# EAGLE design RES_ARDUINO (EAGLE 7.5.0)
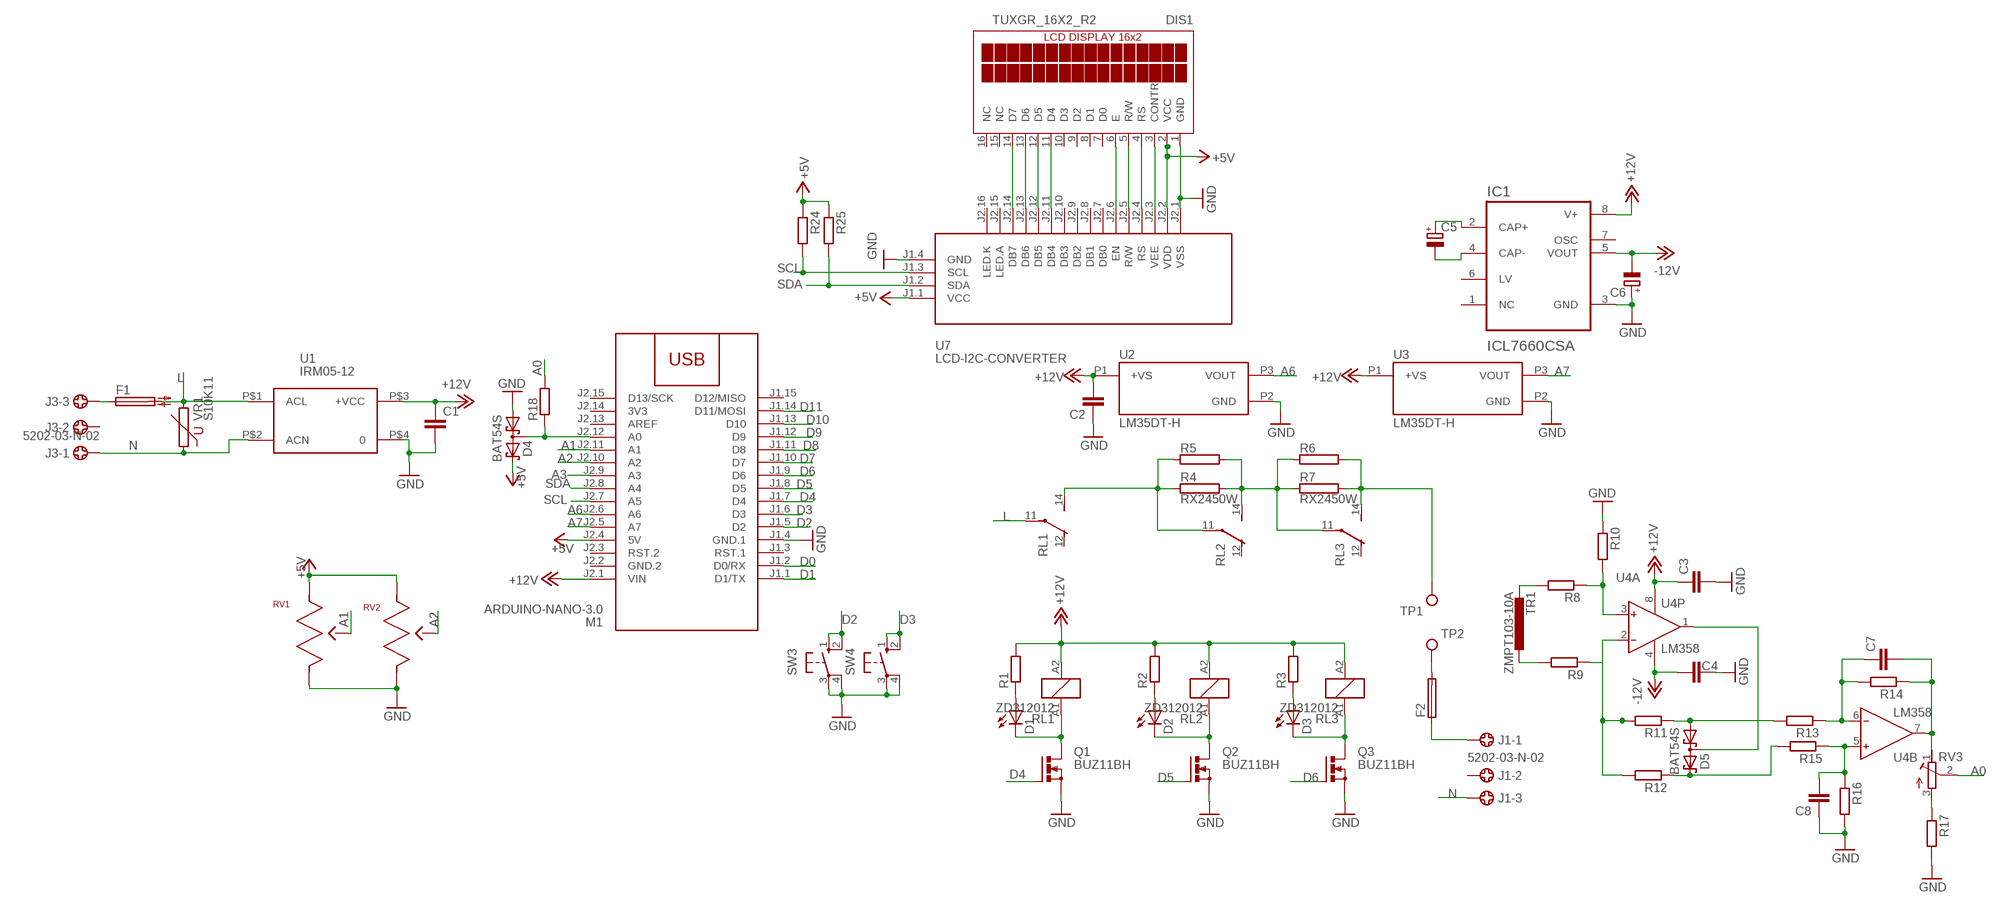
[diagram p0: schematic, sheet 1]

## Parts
C1  C-EUC1206  [C1206]
C2  C-EUC1206  [C1206]
C3  C-EUC1206  [C1206]
C4  C-EUC1206  [C1206]
C5  CPOL-EUSMCB  [SMC_B]
C6  CPOL-EUSMCB  [SMC_B]
C7  C-EUC1206  [C1206]
C8  C-EUC1206  [C1206]
D1  LED5MM  [LED5MM]
D2  LED5MM  [LED5MM]
D3  LED5MM  [LED5MM]
D4  BAT54S  [SOT23]
D5  BAT54S  [SOT23]
DIS1  TUXGR_16X2_R2  [TUXGR_16X2_R2]
F1  SH22,5A  [SH22,5A]
F2  SH22,5A  [SH22,5A]
IC1  ICL7660CSA  [SOIC127P600X175-8N]
J1  5202-03-N-02  [5202-03-N-02]
J3  5202-03-N-02  [5202-03-N-02]
M1  ARDUINO-NANO-3.0  [ARDUINO-NANO-3.0]
Q1  BUZ11BH  [TO220BH]
Q2  BUZ11BH  [TO220BH]
Q3  BUZ11BH  [TO220BH]
R1  R-EU_R1206  [R1206]
R2  R-EU_R1206  [R1206]
R3  R-EU_R1206  [R1206]
R4  RX2450W  [RX2450W]
R5  RX2450W  [RX2450W]
R6  RX2450W  [RX2450W]
R7  RX2450W  [RX2450W]
R8  R-EU_R1206  [R1206]
R9  R-EU_R1206  [R1206]
R10  R-EU_R1206  [R1206]
R11  R-EU_R1206  [R1206]
R12  R-EU_R1206  [R1206]
R13  R-EU_R1206  [R1206]
R14  R-EU_R1206  [R1206]
R15  R-EU_R1206  [R1206]
R16  R-EU_R1206  [R1206]
R17  R-EU_R1206  [R1206]
R18  R-EU_R1206  [R1206]
R24  R-EU_R1206  [R1206]
R25  R-EU_R1206  [R1206]
RL1  ZD312012  [ZD1]
RL2  ZD312012  [ZD1]
RL3  ZD312012  [ZD1]
RV1  PTV09A-4025F-A103  [PTV09]
RV2  PTV09A-4025F-A103  [PTV09]
RV3  R-TRIMM-3386-F  [R-TRIMM-3386F]
SW3  10-XX  [B3F-10XX]
SW4  10-XX  [B3F-10XX]
TP1  TPPAD1-20Y  [P1-20Y]
TP2  TPPAD1-20Y  [P1-20Y]
TR1  ZMPT103-10A  [ZMPT103-10A]
U1  IRM05-12  [IRM05-12]
U2  LM35DT-H  [LM35DT-H]
U3  LM35DT-H  [LM35DT-H]
U4  LM358  AD8042N  [DIL08]
U7  LCD-I2C-CONVERTER  [LCD-I2C-CONVERTER]
VR1  S10K11  [S10K11]

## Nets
+5V: D4.2(C2) DIS1.2(VCC) M1.J2.4(5V) R24.1 R25.1 RV1.1 RV2.1 U7.J1.1(VCC) U7.J2.2(VDD)
+12V: C1.1 C2.2 C3.1 IC1.8(V+) M1.J2.1(VIN) R1.2 R2.2 R3.2 RL1.A2 RL2.A2 RL3.A2 U1.P$3(+VCC) U2.P1(+VS) U3.P1(+VS) U4.8(P:V+)
-12V: C4.1 C6.- IC1.5(VOUT) U4.4(P:V-)
A0: R18.2 RV3.2(S)
A1: M1.J2.11(A1) RV1.2
A2: M1.J2.10(A2) RV2.2
A3: M1.J2.9(A3)
A6: M1.J2.6(A6) U2.P3(VOUT)
A7: M1.J2.5(A7) U3.P3(VOUT)
D0: M1.J1.2(D0/RX)
D1: M1.J1.1(D1/TX)
D2: M1.J1.5(D2) SW3.1(S) SW3.2(S1)
D3: M1.J1.6(D3) SW4.1(S) SW4.2(S1)
D4: M1.J1.7(D4) Q1.G
D5: M1.J1.8(D5) Q2.G
D6: M1.J1.9(D6) Q3.G
D7: M1.J1.10(D7)
D8: M1.J1.11(D8)
D9: M1.J1.12(D9)
D10: M1.J1.13(D10)
D11: M1.J1.14(D11/MOSI)
GND: C1.2 C2.1 C3.2 C4.2 C6.+ C8.1 D4.1(A1) DIS1.1(GND) IC1.3(GND) M1.J1.4(GND.1) Q1.S Q2.S Q3.S R10.1 R16.2 R17.2 RV1.3 RV2.3 SW3.3(P) SW3.4(P1) SW4.3(P) SW4.4(P1) U1.P$4 U2.P2(GND) U3.P2(GND) U7.J1.4(GND) U7.J2.1(VSS)
L: F1.2 RL1.11(2:P) U1.P$1(ACL) VR1.2
N: J1.3 J3.1 U1.P$2(ACN) VR1.1
N$1: DIS1.14(D7) U7.J2.14(DB7)
N$2: DIS1.13(D6) U7.J2.13(DB6)
N$3: DIS1.12(D5) U7.J2.12(DB5)
N$4: DIS1.11(D4) U7.J2.11(DB4)
N$5: DIS1.6(E) U7.J2.6(EN)
N$6: DIS1.5(R/W) U7.J2.5(R/W)
N$7: DIS1.4(RS) U7.J2.4(RS)
N$8: F1.1 J3.3
N$9: D2.A R2.1
N$10: DIS1.3(CONTR) U7.J2.3(VEE)
N$12: D1.K(C) Q1.D RL1.A1
N$13: D2.K(C) Q2.D RL2.A1
N$14: D3.K(C) Q3.D RL3.A1
N$15: R4.P$1 R5.P$1 RL1.14(2:S) RL2.11(2:P)
N$16: R4.P$2 R5.P$2 R6.P$1 R7.P$1 RL2.14(2:S) RL3.11(2:P)
N$17: D1.A R1.1
N$18: D3.A R3.1
N$19: F2.2 TP2.TP
N$20: R6.P$2 R7.P$2 RL3.14(2:S) TP1.TP
N$21: F2.1 J1.1
N$22: R8.2 TR1.P$1
N$23: R9.2 TR1.P$2
N$24: R8.1 R10.2 U4.3(A:IN+)
N$25: C5.+ IC1.2(CAP+)
N$26: C5.- IC1.4(CAP-)
N$27: R9.1 R11.2 R12.2 U4.2(A:IN-)
N$28: D5.1(A1) R11.1 R13.2
N$29: D5.2(C2) R12.1 R15.2
N$30: D5.3(C1A2) U4.1(A:OUT)
N$31: C7.1 R13.1 R14.2 U4.6(B:IN-)
N$32: R17.1 RV3.3(E)
N$33: C8.2 R15.1 R16.1 U4.5(B:IN+)
N$34: D4.3(C1A2) M1.J2.12(A0) R18.1
N$35: C7.2 R14.1 RV3.1(A) U4.7(B:OUT)
SCL: M1.J2.7(A5) R24.2 U7.J1.3(SCL)
SDA: M1.J2.8(A4) R25.2 U7.J1.2(SDA)
Unconnected: DIS1.7(D0) DIS1.8(D1) DIS1.9(D2) DIS1.10(D3) DIS1.15(NC) DIS1.16(NC) IC1.1(NC) IC1.6(LV) IC1.7(OSC) J1.2 J3.2 M1.J1.3(RST.1) M1.J1.15(D12/MISO) M1.J2.3(RST.2) M1.J2.13(AREF) M1.J2.15(D13/SCK) RL1.12(2:O) RL2.12(2:O) RL3.12(2:O) U7.J2.7(DB0) U7.J2.8(DB1) U7.J2.9(DB2) U7.J2.10(DB3) U7.J2.15(LED.A) U7.J2.16(LED.K)

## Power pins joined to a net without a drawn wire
3V3: M1.J2.14(3V3)
GND.2: M1.J2.2(GND.2)

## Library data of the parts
C1-C4 C7 C8 = rcl:C-EU: CAPACITOR, European symbol
C5 C6 = rcl:CPOL-EU: POLARIZED CAPACITOR, European symbol
D1-D3 = led:LED: LED
D4 D5 = diode:BAT54S: Schottky Diodes Pin connection corrected 2011-05-04 Source: Fairchild .. BAT54.pdf
DIS1 = display-lcd:TUXGR_16X2_R2: Tuxgraphics LCD display 16x2 characters reflective, without background light Source: tuxgr_12x2_r2.pdf; OC_FARNELL: unknown; OC_NEWARK: unknown
F1 F2 = fuse:SH22,5A: FUSE HOLDER; MPN: 0031.7701.11; OC_FARNELL: unknown; OC_NEWARK: 04F1224
IC1 = ICL7660CSA:ICL7660CSA: Check availability; AVAILABILITY: In Stock; CHECK_PRICES: https://www.snapeda.com/parts/ICL7660CSA/Analog+Devices/view-part/?ref=eda; DESCRIPTION: Charge Pump Switching Regulator IC Positive or Negative Fixed -Vin, nVin, Vin/2 1 Output 20mA 8-SOIC (0.154, 3.90mm Width); MF: Analog Devices; MP: ICL7660CSA; PACKAGE: SOIC-8 Maxim; PRICE: None; SNAPEDA_LINK: https://www.snapeda.com/parts/ICL7660CSA/Analog+Devices/view-part/?ref=snap
J1 J3 = con-ebyelectro:5202-03-N-02: Barrier Blocks Sreies 5202 Source: http://www.ebyelectro.com/PDF/5202-XX-N-02.pdf; OC_FARNELL: unknown; OC_NEWARK: unknown
M1 = diy-modules:ARDUINO-NANO-3.0: Arduino Nano 3.0 and compatible devices More details available here: https://www.arduino.cc/en/Main/ArduinoBoardNano Click here to find device on ebay.com
Q1-Q3 = transistor-power:BUZ11: N-CHANNEL MOS FET
R1-R3 R8-R18 R24 R25 = rcl:R-EU_: RESISTOR, European symbol
R4-R7 = resistor-power:RX2450W
RL1-RL3 = relay:ZD?1*: Power Relay SCHRACK 1 pole 30 A Source: http://www.schrack.com/.. 5848.pdf; OC_FARNELL: unknown; OC_NEWARK: unknown
RV1 RV2 = PTV09A-4025F-A103:PTV09A-4025F-A103: 10k Ohm 1 Gang Logarithmic Through Hole, Snap In Potentiometer None 1 Turn Carbon 0.05W, 1/20W PC Pins, Board Locks Check availability; AVAILABILITY: In Stock; CHECK_PRICES: https://www.snapeda.com/parts/PTV09A-4025F-A103/Bourns/view-part/?ref=eda; DESCRIPTION: 10k Ohm 1 Gang Logarithmic Through Hole, Snap In Potentiometer None 1.0 Kierros Carbon 0.05W, 1/20W PC Pins, Board Locks; MF: Bourns; MP: PTV09A-4025F-A103; PACKAGE: None; PRICE: None; PURCHASE-URL: https://www.snapeda.com/api/url_track_click_mouser/?unipart_id=1440680&manufacturer=Bourns&part_name=PTV09A-4025F-A103&search_term=ptv09a; SNAPEDA_LINK: https://www.snapeda.com/parts/PTV09A-4025F-A103/Bourns/view-part/?ref=snap
RV3 = rcl:R-TRIMM-3386-F
SW3 SW4 = switch-omron:10-XX: OMRON SWITCH; MPN: B3F-1000; OC_FARNELL: 176432; OC_NEWARK: 36M3542
TP1 TP2 = testpad:TP: Test pad
TR1 = diy-modules:ZMPT103-10A
U1 = acdc:IRM05-12
U2 U3 = LM35DT-H:LM35DT-H
U4 = analog-devices:AD8042: Dual 160 MHz Rail-to-Rail Amplifier Source: http://www.analog.com/static/imported-files/data_sheets/AD8042.pdf; MF: ANALOG DEVICES; MPN: AD8042AN; OC_FARNELL: 1540543; OC_NEWARK: 52F8033
U7 = diy-modules:LCD-I2C-CONVERTER: I2C Bus to 4-Bit Parallel LCD Interface with LED backlight driver
VR1 = varistor:S10K11: VARISTOR

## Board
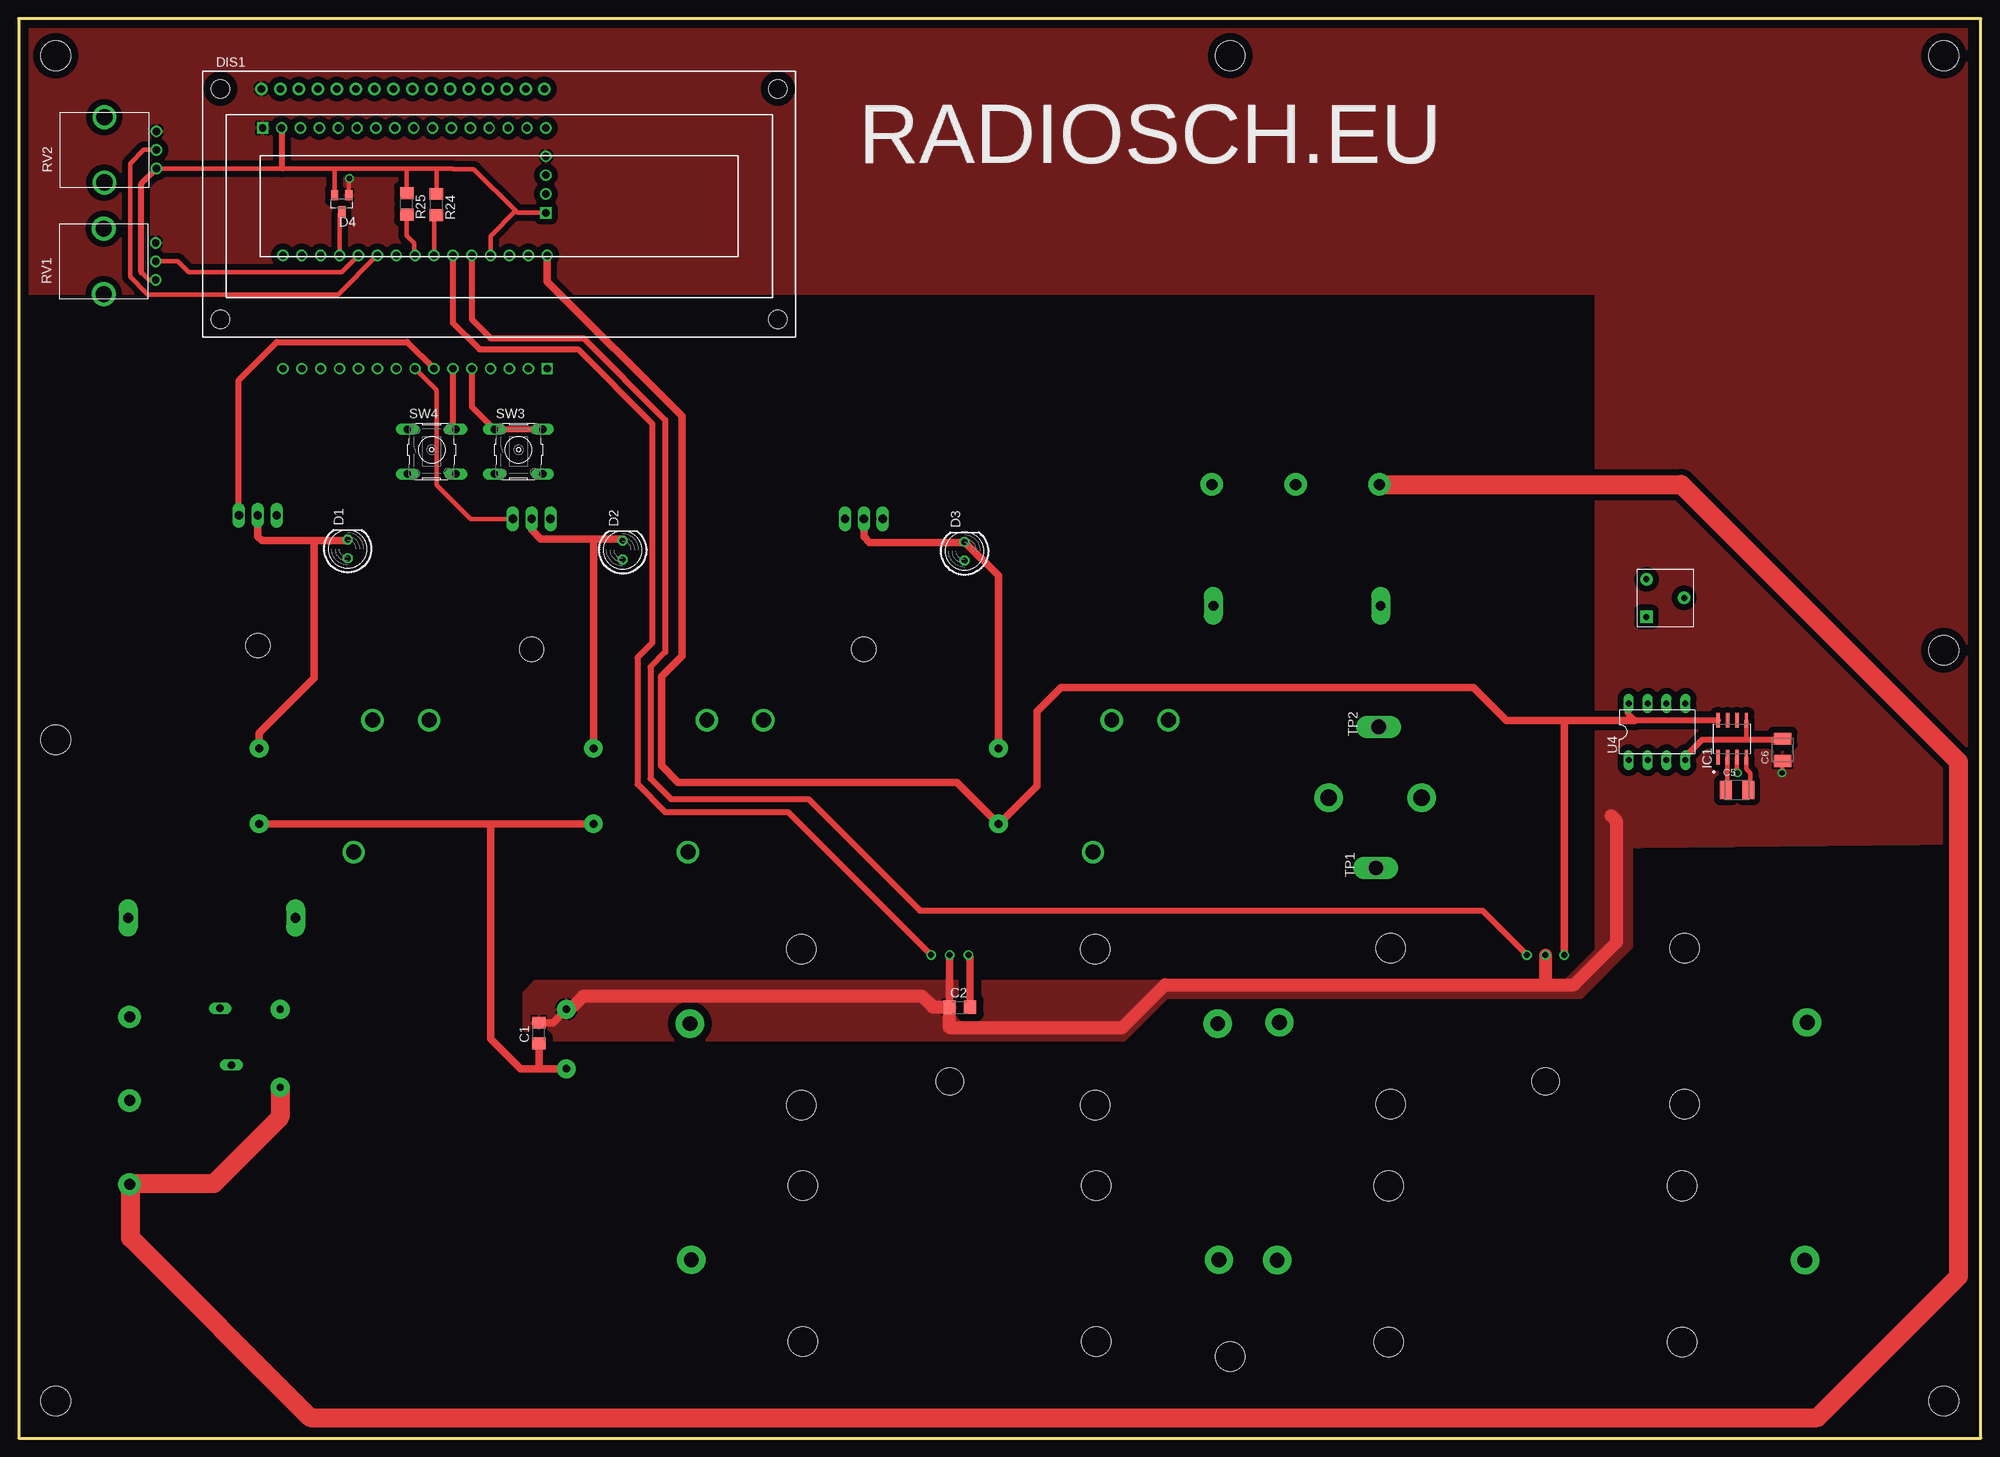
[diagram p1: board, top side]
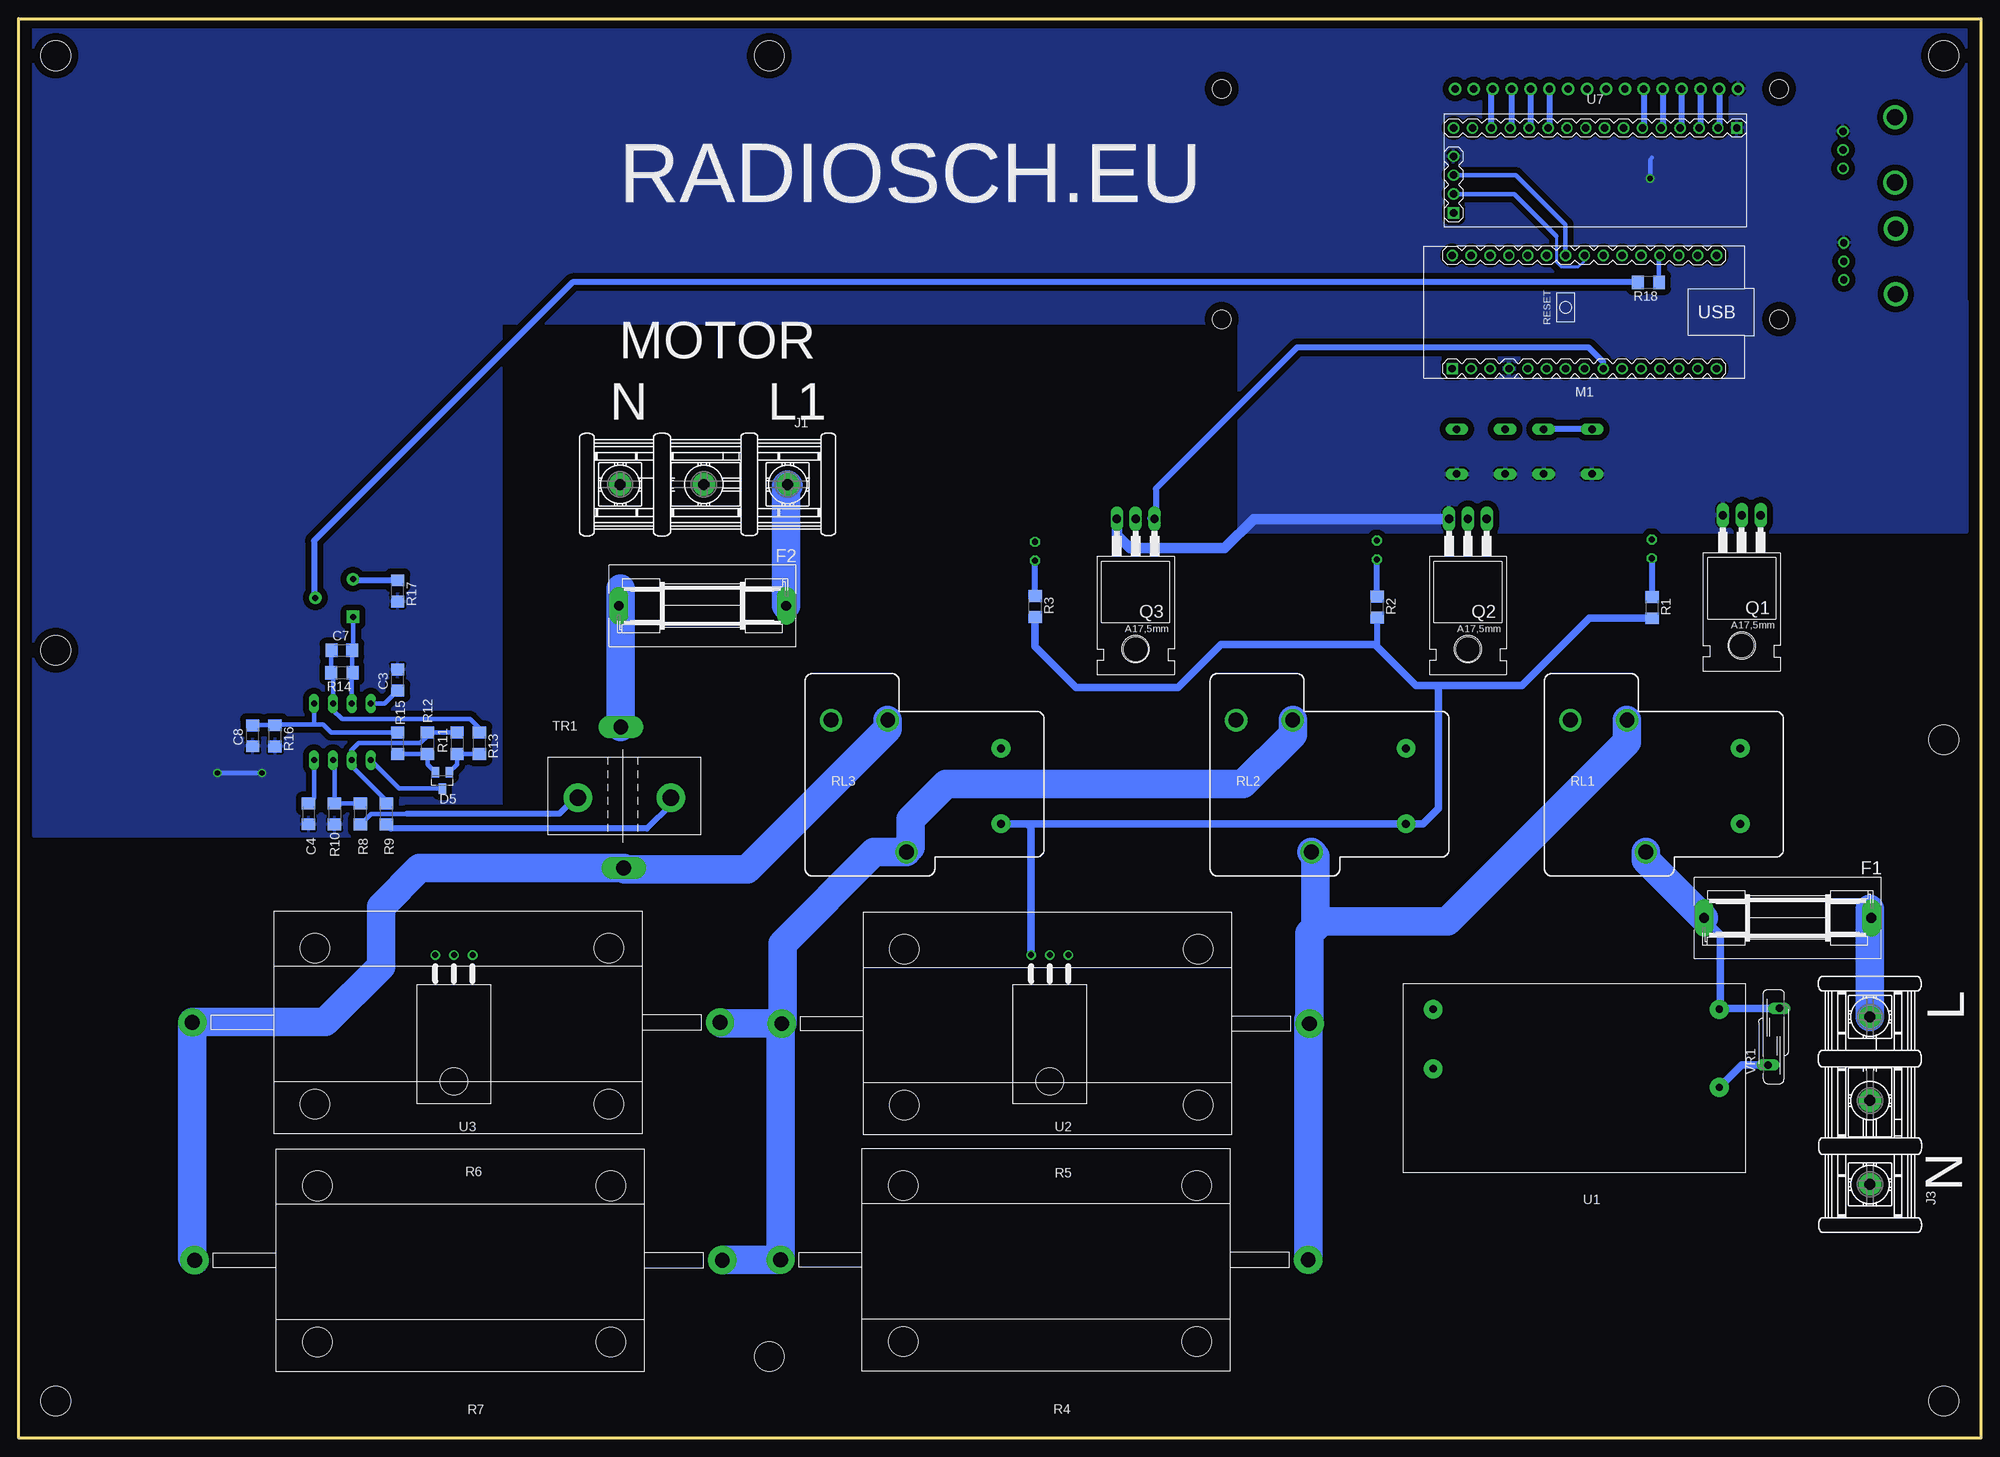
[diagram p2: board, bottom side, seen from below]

Size 264 x 191 mm. Coordinates in mm from the lower left corner, seen from the top.
Outline: 0,0 264,0 264,191 0,191 0,0
Copper layers (1*16): Top 0.035mm / dielectric 1.5mm / Bottom 0.035mm
Design rules "default": minimum track width 10mil, minimum drill 24mil, track to track 8mil, track to pad 8mil, pad to pad 8mil, via to via 8mil, smd to smd 8mil, copper to edge 40mil, drill to drill 8mil, minimum pad ring 10mil, minimum via ring 8mil, stop-mask expansion 4mil, vias tented up to drill 0mil, thermal gap 10mil
Holes 4 mm at 5,186 5,94 5,5 163,11 259,5 259,106 163,186 259,186

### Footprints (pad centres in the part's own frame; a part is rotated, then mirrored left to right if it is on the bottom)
C1206 = smd 1.6 x 1.8: 1 -1.4,0; 2 1.4,0
SMC_B = smd 1.6 x 2.4: + -1.5,0; - 1.5,0
LED5MM = drill 0.813 octagon: A -1.27,0; K 1.27,0
SOT23 = smd 1 x 1.4: 1 -0.95,-1.1; 2 0.95,-1.1; 3 0,1.1
TUXGR_16X2_R2 = drill 1 pad 1.676: 1 -32,15.5; 2 -29.46,15.5; 3 -26.92,15.5; 4 -24.38,15.5; 5 -21.84,15.5; 6 -19.3,15.5; 7 -16.76,15.5; 8 -14.22,15.5; 9 -11.68,15.5; 10 -9.14,15.5; 11 -6.6,15.5; 12 -4.06,15.5; 13 -1.52,15.5; 14 1.02,15.5; 15 3.56,15.5; 16 6.1,15.5 | hole 2.5: -37.5,-15.5; 37.5,-15.5; -37.5,15.5; 37.5,15.5
SH22,5A = drill 1.321 pad 2.54 long: 1 -11.252,0; 2 11.252,0
SOIC127P600X175-8N = smd 1.97 x 0.59: 1 -2.475,1.905; 2 -2.475,0.635; 3 -2.475,-0.635; 4 -2.475,-1.905; 5 2.475,-1.905; 6 2.475,-0.635; 7 2.475,0.635; 8 2.475,1.905
5202-03-N-02 = drill 1.5 pad 3: 1 -9.29,0; 2 2,0; 3 13.25,0
ARDUINO-NANO-3.0 = drill 1 square: J1.1 17.78,7.62 | drill 1: J1.2 15.24,7.62; J1.3 12.7,7.62; J1.4 10.16,7.62; J1.5 7.62,7.62; J1.6 5.08,7.62; J1.7 2.54,7.62; J1.8 0,7.62; J1.9 -2.54,7.62; J1.10 -5.08,7.62; J1.11 -7.62,7.62; J1.12 -10.16,7.62; J1.13 -12.7,7.62; J1.14 -15.24,7.62; J1.15 -17.78,7.62; J2.1 17.78,-7.62; J2.2 15.24,-7.62; J2.3 12.7,-7.62; J2.4 10.16,-7.62; J2.5 7.62,-7.62; J2.6 5.08,-7.62; J2.7 2.54,-7.62; J2.8 0,-7.62; J2.9 -2.54,-7.62; J2.10 -5.08,-7.62; J2.11 -7.62,-7.62; J2.12 -10.16,-7.62; J2.13 -12.7,-7.62; J2.14 -15.24,-7.62; J2.15 -17.78,-7.62
TO220BH = drill 1.118 long: D 0,-6.35; G -2.54,-6.35; S 2.54,-6.35 | hole 3.302: 0,11.176
R1206 = smd 1.6 x 1.803: 1 -1.422,0; 2 1.422,0
RX2450W = drill 2 pad 3.81: P$1 -15,9; P$2 56,9 | hole 4: 0,20; 0,-1; 39.5,-1; 39.5,20
ZD1 = drill 2 pad 2.5: 11 -2.54,-8.88; 12 -12.7,8.88; 14 -5.08,8.88 | drill 1.1 pad 2.5: A1 10.16,5.08; A2 10.16,-5.08
PTV09 = drill 1: 1 -2.5,0; 2 0,0; 3 2.5,0 | drill 2.2: NC1 -4.4,7; NC2 4.4,7
R-TRIMM-3386F = drill 0.8 pad 1.676 square: 1 0,0 | drill 0.8 pad 1.676: 2 5.08,2.54; 3 0,5.08
B3F-10XX = drill 1.016 long: 1 -3.251,2.761; 2 3.251,2.761; 3 -3.251,-3.261; 4 3.251,-3.261
P1-20Y = drill 2.007 pad 2.54 long: TP 0,0
ZMPT103-10A = drill 2.2 pad 3.81: P$1 -1,-5; P$2 11.5,-5
IRM05-12 = drill 1 pad 2.54: P$1 3.5,3.5; P$2 3.5,14; P$3 42,11.5; P$4 42,3.5
LM35DT-H = drill 0.8: P1 2.5,-17; P2 0,-17; P3 -2.5,-17 | hole 3.7: 0,0
DIL08 = drill 0.813 long: 1 -3.81,-3.81; 2 -1.27,-3.81; 3 1.27,-3.81; 4 3.81,-3.81; 5 3.81,3.81; 6 1.27,3.81; 7 -1.27,3.81; 8 -3.81,3.81
LCD-I2C-CONVERTER = drill 1 square: J1.1 -19.05,-5.08; J2.1 19.05,6.35 | drill 1: J1.2 -19.05,-2.54; J1.3 -19.05,0; J1.4 -19.05,2.54; J2.2 16.51,6.35; J2.3 13.97,6.35; J2.4 11.43,6.35; J2.5 8.89,6.35; J2.6 6.35,6.35; J2.7 3.81,6.35; J2.8 1.27,6.35; J2.9 -1.27,6.35; J2.10 -3.81,6.35; J2.11 -6.35,6.35; J2.12 -8.89,6.35; J2.13 -11.43,6.35; J2.14 -13.97,6.35; J2.15 -16.51,6.35; J2.16 -19.05,6.35
S10K11 = drill 1.016 long: 1 -0.762,-3.81; 2 0.762,3.81

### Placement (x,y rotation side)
C1  70,54.5 90 top
C2  126.62,57.97 0 top
C3  213,102 90 bottom
C4  225,84 270 bottom
C5  231.2,87.19 0 top
C6  237.31,92.6 90 top
C7  220.5,106 0 bottom
C8  232.5,94.5 90 bottom
D1  44.28,119.65 90 top
D2  81.28,119.49 90 top
D3  127.28,119.33 90 top
D4  43.47,166.14 180 top
D5  207,88.5 180 bottom
DIS1  64.66,166.05 0 top
F1  26,70 180 bottom
F2  172,112 180 bottom
IC1  230.54,94.09 90 top
J1  169.82,128.32 180 bottom
J3  14.93,43.43 90 bottom
M1  53.34,151.52 180 bottom
Q1  32.18,117.83 180 bottom
Q2  69.02,117.33 180 bottom
Q3  113.72,117.33 180 bottom
R1  44.23,111.74 270 bottom
R2  81.23,111.82 270 bottom
R3  127.23,111.9 270 bottom
R4  105.5,33 180 bottom
R5  105.32,64.78 180 bottom
R6  184.62,64.95 180 bottom
R7  184.32,32.95 180 bottom
R8  218,84 270 bottom
R9  214.5,84 270 bottom
R10  221.5,84 90 bottom
R11  205,93.5 90 bottom
R12  209,93.5 90 bottom
R13  202,93.5 270 bottom
R14  220.5,103 180 bottom
R15  213,93.5 270 bottom
R16  229.5,94.5 270 bottom
R17  213,114 270 bottom
R18  44.72,155.51 180 bottom
R24  56.23,165.98 270 top
R25  52.23,166.06 270 top
RL1  42.53,87.73 0 bottom
RL2  87.51,87.73 0 bottom
RL3  141.99,87.73 0 bottom
RV1  18.45,158.33 90 top
RV2  18.55,173.33 90 top
RV3  219,110.5 0 top
SW3  67.26,132.99 0 top
SW4  55.58,132.99 0 top
TP1  182.59,76.71 90 top
TP2  182.98,95.71 90 top
TR1  187.75,91.15 0 bottom
U1  31.69,61.2 180 bottom
U2  125.27,48 180 bottom
U3  205.43,48 180 bottom
U4  220.43,95.03 0 top
U7  51.89,169.94 0 bottom
VR1  27.88,54.03 0 bottom

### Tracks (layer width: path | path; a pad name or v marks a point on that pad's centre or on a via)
+5V
  Top 0.61: RV2.1 35.5,170.83 42.25,170.83 | 42.25,170.83 52,170.83 | 52,170.83 56.25,170.83 | 56.25,170.83 58.42,170.83 58.5,170.75 61.25,170.75 66.88,165.12 | R25.1 52.23,170.6 52,170.83 | R24.1 56.23,170.81 56.25,170.83 | D4.2 42.52,170.56 42.25,170.83 | U7.J1.1 67.14,164.86 66.88,165.12 | M1.J2.4 63.5,161.75 66.88,165.12 | RV1.1 17.55,155.83 16.5,156.88
  Top 0.813: 16.5,156.88 16.5,168.78 RV2.1 | U7.J2.2 35.38,170.95 35.5,170.83
  Bottom 0.813: DIS1.2 35.2,176.47 U7.J2.2
+12V
  Top 0.813: IC1.8 217.44,96.56 216.5,97.5 216.5,98.72 U4.8
  Top 1.016: M1.J2.1 71.12,155.63 89.25,137.5 89.25,105.25 86.5,102.5 86.5,90.5 88.75,88.25 126.23,88.25 RL3.A2 131.9,82.65 137,87.75 137,97.75 140.25,101 195.75,101 200.19,96.56 208,96.56 | RL1.A2 63.25,82.65 | 63.25,82.65 RL2.A2 | C2.2 128.02,64.75 U2.P1 | U1.P$3 70.25,49.7 | 70.25,49.7 67.55,49.7 63.5,53.75 63.5,82.4 63.25,82.65 | C1.1 70,49.95 70.25,49.7 | 217.44,96.56 208,96.56 | U3.P1 207.93,96.5 208,96.56
  Bottom 0.61: U4.8 214.76,98.84 C3.1
  Bottom 0.813: R2.2 81.23,106.52 81.25,106.5
  Bottom 1.016: R1.2 52.68,110.32 61.75,101.25 73,101.25 | 73,101.25 76,101.25 81.25,106.5 81.5,106.75 102.25,106.75 108,101 121.75,101 127.25,106.5 127.25,110.46 R3.2 | 128.25,82.65 RL2.A2 75.1,82.65 73,84.75 73,101.25 | 128.25,82.65 RL3.A2 | U2.P1 127.77,82.17 128.25,82.65
-12V
  Top 0.61: IC1.5 232.44,94.06 232.5,94
  Top 0.813: U4.4 224.24,91.74 226.5,94 232.5,94 237.21,94 C6.-
  Bottom 0.61: U4.4 224.24,86.16 C4.1
A0
  Bottom 0.813: RV3.2 224.25,113.21 224.25,120.75 189.49,155.51 R18.2
A1
  Top 0.61: RV1.2 21.42,158.33 22.88,156.88 43.45,156.88 M1.J2.11
A2
  Top 0.61: RV2.2 16.83,173.33 15,171.5 15,156.25 17.38,153.88 42.99,153.88 M1.J2.10
A6
  Top 0.813: M1.J2.6 58.42,150.08 62,146.5 75.25,146.5 85.25,136.5 85.25,107 83.25,105 83.25,88 87,84.25 103.52,84.25 U2.P3
A7
  Top 0.813: M1.J2.5 60.96,150.54 63.5,148 76,148 87,137 87,105.75 85,103.75 85,88.75 87.75,86 106.25,86 121.25,71 196.93,71 U3.P3
D2
  Top 0.813: M1.J1.5 60.96,138.8 SW3.1 SW3.2
D3
  Top 0.813: M1.J1.6 58.42,136.16 SW4.2
  Bottom 0.813: SW4.1 SW4.2
D4
  Top 0.813: Q1.G 29.64,142.39 34.75,147.5 52.28,147.5 M1.J1.7
D5
  Top 0.61: Q2.G 60.82,123.68 56.25,128.25 56.25,140.99 M1.J1.8
D6
  Bottom 0.813: M1.J1.9 50.8,144.8 52.75,146.75 92,146.75 111,127.75 111,124.5 111.75,123.75 111.25,123.75 Q3.G
GND  (via drill 0.7)
  Top 0.61: IC1.3 231.18,89.58 v231.25,89.5 | v237.25,89.5 C6.+ | D4.1 44.42,169.42 v44.5,169.5
  Top 1.016: U1.P$4 71.89,55.9 C1.2 | C2.1 125.22,64.95 U2.P2
  Top 1.778: 125.19,58 125.19,55.31 125.25,55.25 148.5,55.25 154.25,61 205,61 | 205,61 209.25,61 215,66.75 215,83 214.25,83.75 | U3.P2 205.43,61.43 205,61 | U1.P$4 74.2,57.7 76,59.5 121.5,59.5 123,58 125.19,58 | 125.19,58 C2.1
  Bottom 0.61: v231.25,89.5 v237.25,89.5 | v44.5,169.5 44.5,172 44.25,172.25
  Bottom 1.422: Q2.S 97.82,123.68 101.75,119.75 114.5,119.75 116.25,121.5 Q3.S
  pour Bottom (isolate 0.813): 2,190 262,190 262,81 199,81 199,150 2,150
  pour Bottom (isolate 0.813): 2,153 99.75,153 99.75,122 2,122
  pour Top (isolate 0.813): 1,190 262,190 262,80 212.25,79.5 212.25,154 1,154
  pour Top (isolate 1.016): 69.5,61.5 208,61.5 212.25,65.75 212.25,80.25 212.5,80.5 216.75,80.5 217,80.25 217,66 210.25,59.25 154.5,59.25 148.75,53.5 69.5,53.5 68,55 68,60
L
  Bottom 1.016: VR1.2 35.05,57.84 | 35.05,57.84 U1.P$1 | 35.05,57.84 35.05,67.8 F1.2
  Bottom 3.81: RL1.11 45.07,77.82 F1.2
N
  Top 2.54: U1.P$2 35.19,43.19 26.25,34.25 15.04,34.25 J3.1 15.07,34 15.07,26.93 39.25,2.75 242,2.75 261,21.75 261,91 223.68,128.32 J1.3
  Bottom 1.016: VR1.1 32.17,50.22 U1.P$2
N$1
  Bottom 0.813: U7.J2.14 65.86,181.37 DIS1.14
N$2
  Bottom 0.813: DIS1.13 63.14,176.47 U7.J2.13
N$3
  Bottom 0.813: DIS1.12 60.6,176.47 U7.J2.12
N$4
  Bottom 0.813: DIS1.11 58.06,176.47 U7.J2.11
N$5
  Bottom 0.813: DIS1.6 45.36,176.47 U7.J2.6
N$6
  Bottom 0.813: DIS1.5 42.82,176.47 U7.J2.5
N$7
  Bottom 0.813: DIS1.4 40.28,176.47 U7.J2.4
N$8
  Bottom 1.422: F1.1 14.75,70.82 14.93,71
  Bottom 3.81: J3.3 14.93,71 14.93,71.23
N$9
  Bottom 0.813: R2.1 81.23,118.17 D2.A
N$10
  Bottom 0.813: DIS1.3 37.74,176.47 U7.J2.3
N$12
  Top 1.016: Q1.D 32.18,121.32 32.75,120.75 39.5,120.75 | 39.5,120.75 44.11,120.75 D1.K | RL1.A1 32.37,94.87 39.75,102.25 39.75,120.5 39.5,120.75
N$13
  Top 1.016: Q2.D 69.02,122.23 70.25,121 77.5,121 | 77.5,121 81.04,121 D2.K | RL2.A1 77.35,120.85 77.5,121
N$14
  Top 1.016: Q3.D 113.72,121.28 114.5,120.5 127.18,120.5 D3.K 131.83,116.05 RL3.A1
N$15
  Bottom 3.81: RL1.14 47.61,93.64 71.75,69.5 88.75,69.5 | 88.75,69.5 89.5,69.5 89.5,78.25 89.75,78.5 89.75,78.55 RL2.11 | R5.P$1 90.32,56.5 | 90.32,56.5 90.32,67.93 88.75,69.5 | R4.P$1 90.5,56.32 90.32,56.5
N$16
  Bottom 0.813: RL3.11 144.53,78.97 144.25,79.25
  Bottom 3.81: RL2.14 92.59,94.66 99.25,88 139.25,88 144,83.25 144,79.5 144.25,79.25 | RL3.11 148.9,78.85 161.25,66.5 161.25,55.85 R5.P$2 162,55.78 | 162,55.78 169.45,55.78 R6.P$1 | R7.P$1 169.27,24 R4.P$2 161.5,56.25 161.53,56.25 162,55.78
N$17
  Bottom 0.813: R1.1 44.23,118.33 D1.A
N$18
  Bottom 0.813: R3.1 127.23,118.01 D3.A
N$19
  Bottom 1.016: 182.98,114.31 182.98,112.27 F2.2
  Bottom 3.81: TP2.TP 182.98,114.31
N$20
  Bottom 3.81: RL3.14 147.07,95.43 166,76.5 182.38,76.5 TP1.TP 210.04,76.71 215.25,71.5 215.25,63.5 222.75,56 240.57,56 R6.P$2 240.62,24.25 R7.P$2
N$21
  Bottom 3.81: 160.39,128.18 J1.1 160.75,128.1 F2.1
N$22
  Bottom 0.61: 211.75,84 216.58,84 R8.2
  Bottom 0.813: TR1.P$1 189.1,86.15 191.25,84 211.75,84
N$23
  Bottom 0.813: TR1.P$2 176.25,85.25 179.5,82 213.92,82 R9.2
N$24
  Bottom 0.61: R8.1 R10.2 221.5,91.02 U4.3
N$25
  Top 0.61: IC1.2 229.91,87.39 C5.+
N$26
  Top 0.61: IC1.4 232.44,90.06 233,89.5 233,87.49 C5.-
N$27
  Bottom 0.61: R11.2 R12.2 209,94.5 210,93.5 218.25,93.5 219.25,92.5 219.25,91.31 U4.2 219.25,91.13 219.25,90.5 214.5,85.75 R9.1
N$28
  Bottom 0.61: R13.2 R11.1 205,90.65 D5.1
N$29
  Bottom 0.61: D5.2 209,90.65 R12.1 R15.2
N$30
  Bottom 0.61: D5.3 212.8,87.4 U4.1
N$31
  Bottom 0.61: R13.1 202,95.5 203.25,96.75 220.5,96.75 221.75,98 221.75,98.79 U4.6 221.7,102.78 R14.2 221.92,105.98 C7.1
N$32
  Bottom 0.813: R17.1 218.84,115.42 RV3.3
N$33
  Bottom 0.61: R15.1 221.92,94.92 223,96 224.25,96 | 224.25,96 229.42,96 R16.1 232.48,95.92 C8.2 | U4.5 224.24,96.01 224.25,96
N$34
  Top 0.61: M1.J2.12 43.18,164.75 D4.3
  Bottom 0.61: R18.1 43.3,159.02 M1.J2.12
N$35
  Bottom 0.61: RV3.1 219,106.1 C7.2 219.1,103.02 R14.1 219.16,102.92 U4.7
SCL
  Top 0.61: M1.J2.7 55.88,164.21 R24.2
  Bottom 0.61: U7.J1.3 62.57,169.94 55.88,163.25 M1.J2.7
SDA
  Top 0.61: R25.2 52.23,161.77 53.25,160.75 53.25,159.23 M1.J2.8
  Bottom 0.406: 57.12,161.75 57.12,158.25 56.5,157.62 54.12,157.62 53.38,158.38 53.38,159.1 M1.J2.8
  Bottom 0.61: U7.J1.2 62.77,167.4 57.12,161.75

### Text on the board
tPlace: RADIOSCH.EU
bPlace: RADIOSCH.EU | MOTOR | L1 | N | L | N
